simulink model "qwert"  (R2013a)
settings: Solver=ode45  StartTime=0.0  StopTime=10.0  RelTol=1e-3

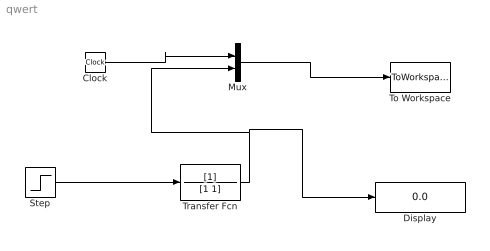
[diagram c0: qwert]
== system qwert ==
  Clock : Clock
  Display : Display
  Mux : Mux  Inputs=2
  Step : Step  Time=0  After=5  SampleTime=0
  To Workspace : ToWorkspace  VariableName=simout  SampleTime=-1
  Transfer Fcn : TransferFcn  Denominator=[1 1]
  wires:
  Step/1 -> Transfer Fcn/1
  Transfer Fcn/1 -> Mux/2, Display/1
  Clock/1 -> Mux/1
  Mux/1 -> To Workspace/1
